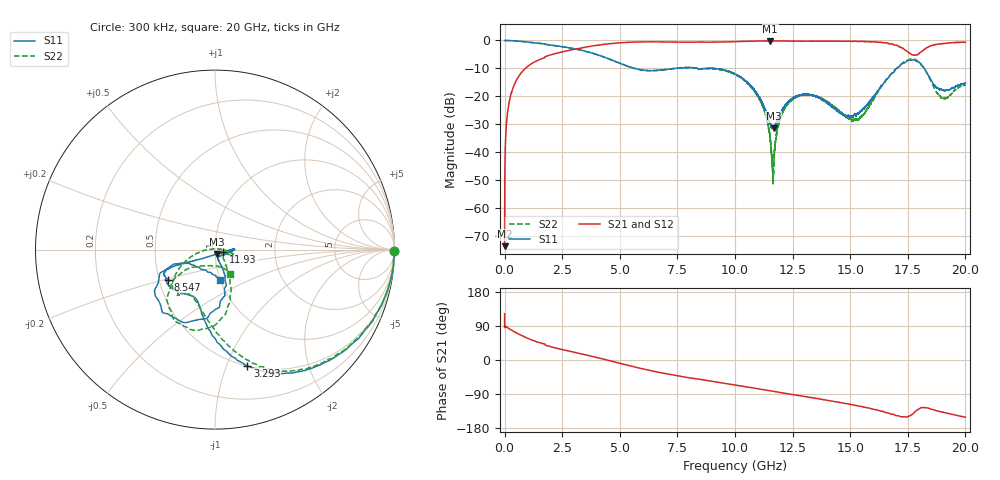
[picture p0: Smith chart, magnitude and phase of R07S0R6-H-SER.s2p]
!{R07S0R6}
!Johanson Technology Inc.
!www.johansontechnology.com
!Test Board Conditions:
!Substrate Type  RO4350B
!Substrate Thickness  10 mil
!Substrate Dk  3.66
!TL Type: GCPW
!TL Trace Width  21 mil
!TL Gap  20 mil
!Electrode orientation  Horizontal
!DUT TOPOLOGY	SERIES
!Mounting Pad LxW  16x21 mil
! Created Fri Feb  5 23:03:38 2021
# hz S ma R 50
! 2 Port Network Data from SP1.SP block
! freq  magS11  angS11  magS21  angS21  magS12  angS12  magS22  angS22
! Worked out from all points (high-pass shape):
!   20001 points, 300 kHz to 20 GHz, reference 50 ohm
!   highest |S21| = -0.15 dB at 11.52 GHz (marker M1); lowest = -73.6 dB at 300 kHz (marker M2)
!   |S21| within 3 dB of the highest: 3.046 GHz to 17.34 GHz (14.29 GHz wide, 140 % of centre); 18.23 GHz to end of sweep
!   lowest |S11| = -31.5 dB at 11.68 GHz (marker M3), VSWR 1.05, Z = 51.2 - j2.43 ohm
!   |S11| at or under -10 dB: 5.652 GHz to 7.456 GHz (1.804 GHz wide, 27.5 % of centre); 9.101 GHz to 17 GHz (7.901 GHz wide, 60.5 % of centre); 18.22 GHz to end of sweep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
!   |S22| runs from -51.8 to 0.0 dB; largest |S21 - S12| = 0.013
!   S11 on the Smith chart (normalised r, x): 300 kHz: open; 3.293 GHz: 0.50, -1.19; 8.547 GHz: 0.56, -0.21; 11.93 GHz: 1.09, -0.03; 20 GHz: 1.00, -0.35
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300000  0.9994 -0.6  0.0002084 122.0  0.0001342 112.6  0.9999 -0.5
1.013e8  0.9971 -3.7  0.04054 86.2  0.0405 86.3  0.9975 -3.6
1.323e8  0.9985 -4.8  0.05294 84.9  0.05278 85.1  0.9981 -4.8
4.943e8  0.9795 -17.4  0.188 72.3  0.1875 72.2  0.9798 -17.1
1.8503e9  0.8426 -52.6  0.5287 37.5  0.5274 37.6  0.8409 -51.6
3.2933e9  0.6722 -74.4  0.729 16.6  0.7291 16.6  0.6701 -71.3
3.3343e9  0.6672 -75.0  0.7369 16.0  0.7353 16.0  0.6666 -71.8
6.6673e9  0.2924 -120.2  0.9444 -32.2  0.9444 -32.2  0.2927 -123.9
8.5473e9  0.3121 -147.7  0.9335 -51.8  0.9362 -51.7  0.3101 -135.7
1.00003e10  0.2535 -157.9  0.9516 -65.9  0.9534 -65.9  0.246 -149.9
1.10413e10  0.09822 -148.0  0.9782 -76.3  0.9781 -76.2  0.0917 -170.3
1.15213e10  0.03215 -106.2  0.9823 -81.2  0.9807 -81.2  0.01859 173.3
1.16763e10  0.02661 -62.9  0.9796 -82.9  0.9798 -82.8  0.005279 44.7
1.19303e10  0.04653 -18.7  0.9774 -85.4  0.9794 -85.5  0.03667 1.2
1.24533e10  0.08886 -0.5  0.973 -90.7  0.975 -90.7  0.08541 -9.2
1.33343e10  0.1056 -1.9  0.9703 -99.4  0.9721 -99.4  0.1059 -19.4
1.53213e10  0.0491 -72.8  0.9613 -120.8  0.9616 -120.9  0.03789 -23.0
1.66673e10  0.2156 -74.3  0.8784 -139.9  0.8831 -140.4  0.2234 -66.9
1.74813e10  0.4331 -110.8  0.6339 -149.9  0.6358 -149.7  0.4435 -96.5
1.79723e10  0.409 -145.4  0.5757 -129.5  0.5795 -129.5  0.4118 -128.4
1.90033e10  0.1302 -120.4  0.8776 -137.4  0.8777 -137.6  0.09314 -104.4
2e10  0.1714 -79.9  0.9321 -151.0  0.9294 -150.9  0.1605 -59.4
